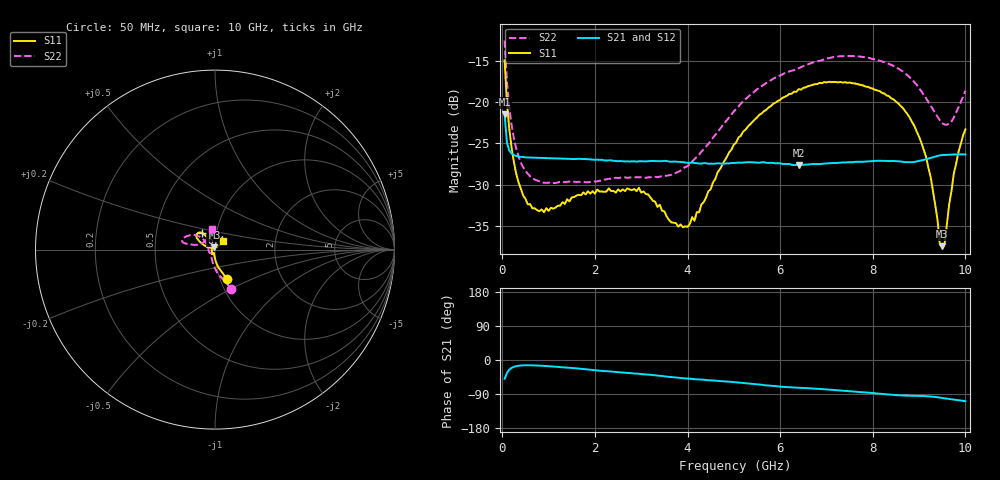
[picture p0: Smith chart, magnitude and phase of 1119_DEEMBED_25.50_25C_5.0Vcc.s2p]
!Hittite Microwave Corp.
!Digital Attenuator/PhaseShifter Rev 1.4.0
!Filename: C:\DATA\DATA\1119_DEEMBED_25.50_25C_5.0Vcc.s2p
!VNA ID: Agilent Technologies,N5224A,MY51441122,A.10.45.03
!Device type:
!2 Port Calibration.
!Temp(C): 25
!Lot Number:
!Serial Number:
!Operator:
!Misc:
!Attenuator:  25.500
# GHZ S DB R 50.0
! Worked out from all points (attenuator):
!   200 points, 50 MHz to 10 GHz, reference 50 ohm
!   highest |S21| = -21.50 dB at 50 MHz (marker M1); lowest = -27.6 dB at 6.4 GHz (marker M2)
!   lowest |S11| = -37.4 dB at 9.5 GHz (marker M3), VSWR 1.03, Z = 49.7 + j1.29 ohm
!   |S11| at or under -10 dB: start of sweep to end of sweep
!   |S22| runs from -29.8 to -12.6 dB; largest |S21 - S12| = 0.00014
!   S11 on the Smith chart (normalised r, x): 50 MHz: 1.08, -0.37; 6.4 GHz: 0.85, +0.16; 10 GHz: 1.09, +0.11
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0.05  -14.96 -67.7  -21.50 -49.7  -21.51 -49.7  -12.56 -67.3
0.1  -20.06 -79.6  -24.90 -34.4  -24.89 -34.5  -17.51 -83.9
0.2  -25.51 -89.2  -26.22 -20.9  -26.23 -20.9  -22.79 -100.5
0.35  -29.69 -96.2  -26.59 -15.2  -26.58 -15.2  -26.57 -114.6
0.55  -32.36 -104.1  -26.70 -13.8  -26.70 -13.9  -28.66 -126.3
0.9  -33.32 -111.1  -26.78 -15.5  -26.78 -15.5  -29.76 -135.7
1.75  -30.92 -122.0  -26.89 -23.9  -26.89 -23.9  -29.66 -140.6
2.95  -30.36 -124.1  -27.15 -36.3  -27.16 -36.4  -29.10 -159.8
3.4  -32.42 -140.1  -27.14 -41.6  -27.15 -41.7  -29.02 -173.4
4  -35.08 167.5  -27.34 -49.0  -27.34 -49.0  -27.75 162.2
5.05  -24.91 122.1  -27.35 -58.8  -27.37 -58.9  -20.83 138.8
6.4  -18.44 128.5  -27.63 -73.1  -27.65 -73.2  -15.92 150.0
6.7  -17.93 132.2  -27.50 -75.2  -27.51 -75.2  -15.24 154.0
8.35  -19.30 150.0  -27.14 -91.0  -27.14 -91.0  -15.39 168.1
8.75  -21.48 154.7  -27.27 -94.1  -27.27 -94.1  -16.76 168.1
9.05  -24.93 159.6  -27.05 -94.8  -27.07 -94.8  -18.71 166.9
9.25  -29.06 159.4  -26.75 -96.4  -26.76 -96.3  -20.44 162.2
9.45  -37.26 127.7  -26.44 -99.3  -26.46 -99.3  -22.23 149.3
9.5  -37.42 104.3  -26.41 -100.3  -26.43 -100.3  -22.57 143.9
9.55  -37.15 75.8  -26.39 -101.2  -26.40 -101.2  -22.72 138.1
9.75  -28.64 44.5  -26.34 -104.4  -26.35 -104.4  -21.88 114.3
10  -23.30 46.2  -26.35 -108.7  -26.35 -108.8  -18.65 98.5
